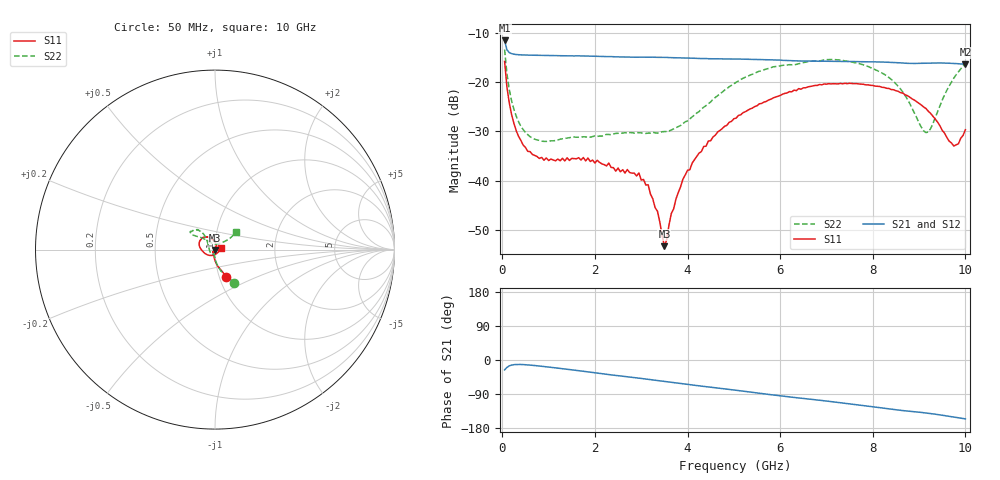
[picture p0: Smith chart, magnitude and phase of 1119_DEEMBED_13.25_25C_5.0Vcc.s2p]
!Hittite Microwave Corp.
!Digital Attenuator/PhaseShifter Rev 1.4.0
!Filename: C:\DATA\DATA\1119_DEEMBED_13.25_25C_5.0Vcc.s2p
!VNA ID: Agilent Technologies,N5224A,MY51441122,A.10.45.03
!Device type:
!2 Port Calibration.
!Temp(C): 25
!Lot Number:
!Serial Number:
!Operator:
!Misc:
!Attenuator:  13.250
# GHZ S DB R 50.0
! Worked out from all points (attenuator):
!   200 points, 50 MHz to 10 GHz, reference 50 ohm
!   highest |S21| = -11.50 dB at 50 MHz (marker M1); lowest = -16.4 dB at 10 GHz (marker M2)
!   lowest |S11| = -53.3 dB at 3.5 GHz (marker M3), VSWR 1.00, Z = 50.2 - j0.138 ohm
!   |S11| at or under -10 dB: start of sweep to end of sweep
!   |S22| runs from -32.0 to -13.3 dB; largest |S21 - S12| = 0.00062
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0.05  -15.77 -67.2  -11.50 -26.1  -11.50 -26.1  -13.34 -59.9
0.1  -20.95 -82.1  -13.40 -19.6  -13.40 -19.5  -18.24 -74.9
0.2  -26.53 -95.1  -14.18 -13.4  -14.19 -13.4  -23.74 -86.3
0.35  -30.97 -106.3  -14.40 -11.8  -14.41 -11.8  -28.00 -93.1
0.55  -34.03 -118.8  -14.48 -12.9  -14.48 -12.9  -30.65 -99.2
0.9  -35.84 -129.7  -14.54 -17.2  -14.54 -17.2  -32.01 -105.4
1.75  -35.29 -134.7  -14.65 -29.8  -14.65 -29.8  -31.08 -115.3
2.95  -38.44 -105.3  -14.89 -47.8  -14.90 -47.9  -30.26 -152.6
3.15  -40.85 -94.3  -14.91 -50.9  -14.92 -51.0  -30.33 -162.8
3.4  -48.34 -83.9  -14.93 -54.9  -14.93 -54.9  -30.21 -175.0
3.5  -53.31 -39.5  -14.93 -56.5  -14.94 -56.6  -30.01 179.1
3.65  -46.67 29.0  -14.99 -58.9  -15.00 -58.9  -29.70 171.3
4  -37.88 57.1  -15.09 -64.4  -15.10 -64.5  -27.84 151.4
4.45  -31.93 70.9  -15.21 -71.2  -15.22 -71.3  -24.34 134.5
5.05  -27.28 89.9  -15.28 -79.9  -15.30 -79.9  -20.01 126.5
6.7  -20.76 131.1  -15.69 -104.1  -15.70 -104.2  -15.69 139.7
7.65  -20.27 154.7  -15.80 -118.0  -15.81 -118.1  -16.06 147.1
8.35  -21.26 170.1  -15.94 -128.9  -15.94 -128.9  -19.04 140.8
8.65  -22.21 179.8  -16.09 -133.6  -16.09 -133.6  -22.00 133.9
9.15  -25.34 -149.4  -16.12 -139.8  -16.14 -139.8  -30.23 90.4
9.75  -32.96 -49.3  -16.17 -150.6  -16.18 -150.5  -19.16 37.3
10  -29.64 12.7  -16.35 -155.4  -16.35 -155.4  -16.23 39.4
